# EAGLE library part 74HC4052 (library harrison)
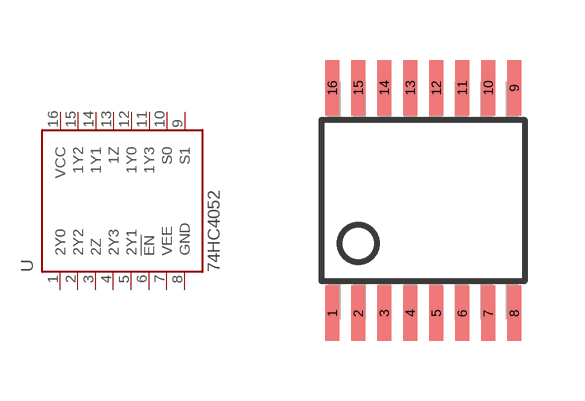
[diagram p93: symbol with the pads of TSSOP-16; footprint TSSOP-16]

Designator prefix U

## 74HC4052_TSSOP-16  [TSSOP-16]
1  2Y0
2  2Y2
3  2Z
4  2Y3
5  2Y1
6  !EN!  in
7  VEE  pwr
8  GND  pwr
9  S1  in
10  S0  in
11  1Y3  in
12  1Y0
13  1Z
14  1Y1
15  1Y2
16  VCC  pwr

## Footprint TSSOP-16 (pad centres in mm)
smd 0.348 x 1.397: 1 -2.273,-2.814; 2 -1.623,-2.815; 3 -0.973,-2.815; 4 -0.323,-2.815; 5 0.327,-2.815; 6 0.977,-2.815; 7 1.627,-2.815; 8 2.277,-2.815; 9 2.277,2.825; 10 1.627,2.825; 11 0.977,2.825; 12 0.327,2.825; 13 -0.323,2.825; 14 -0.973,2.825; 15 -1.623,2.825; 16 -2.273,2.825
